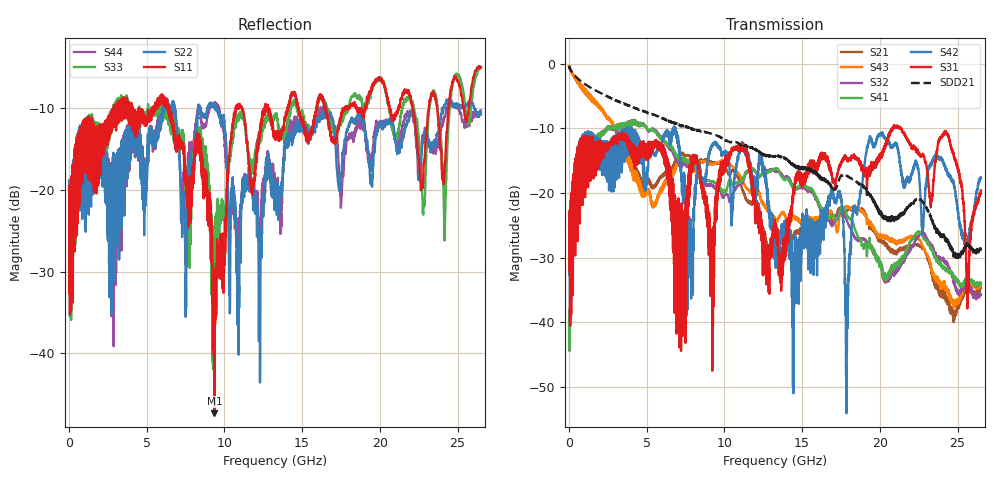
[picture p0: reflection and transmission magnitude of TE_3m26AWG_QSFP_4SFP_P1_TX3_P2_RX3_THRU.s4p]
! Touchstone data
! Created: 03-Feb-2015 by IdEM R2012 (8.0.5)
# Hz S MA R 50
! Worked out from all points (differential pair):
!   2650 points, 10 MHz to 26.5 GHz, reference 50 ohm
!   strongest paths, dB at 10 MHz, 6.63 GHz, 13.26 GHz, 19.88 GHz, 26.5 GHz:
!     S31: -25.0, -17.8, -24.8, -15.3, -19.6
!     S42: -25.1, -10.7, -28.5, -11.1, -17.6
!     S41: -40.5, -13.1, -16.2, -29.9, -34.0
!     S32: -40.6, -13.5, -16.6, -29.9, -35.7
!     S43: -0.3, -16.9, -23.8, -26.6, -34.3
!     S21: -0.4, -16.0, -26.9, -27.1, -34.7
!   taken as a pair (ports 3,1 in; 4,2 out), SDD21 dB: -0.3, -9.0, -14.3, -22.4, -28.7
!   lowest |S11| = -47.3 dB at 9.36 GHz (marker M1), VSWR 1.01, Z = 50.3 + j0.257 ohm
!   |S11| at or under -10 dB: start of sweep to 2.897 GHz; 6.442 GHz to 10.73 GHz (4.284 GHz wide, 49.9 % of centre); 11.14 GHz to 12.6 GHz (1.454 GHz wide, 12.2 % of centre)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
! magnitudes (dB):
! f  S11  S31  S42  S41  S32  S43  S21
! 10 MHz  -19.6  -25.0  -25.1  -40.5  -40.6  -0.3  -0.4
! 1.99 GHz  -15.4  -14.1  -13.5  -11.3  -11.3  -6.6  -6.5
! 9.36 GHz  -47.3  -27.5  -12.3  -18.3  -19.0  -15.4  -15.4
! 10.85 GHz  -10.1  -12.6  -14.7  -18.4  -18.9  -16.8  -17.4
! 17.87 GHz  -10.0  -14.9  -43.0  -23.3  -24.2  -22.1  -22.8
! 19.35 GHz  -8.3  -16.8  -11.4  -27.1  -27.5  -24.8  -25.5
! 26.5 GHz  -5.0  -19.6  -17.6  -34.0  -35.7  -34.3  -34.7
